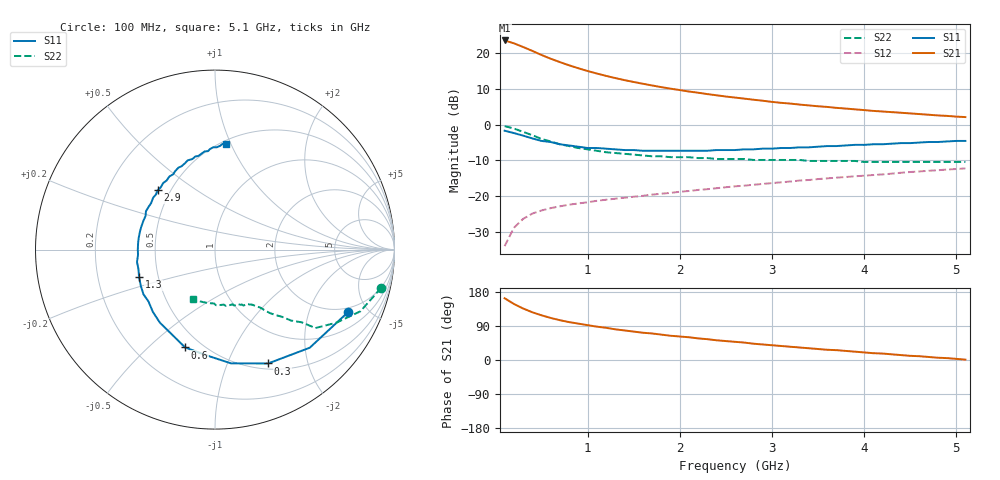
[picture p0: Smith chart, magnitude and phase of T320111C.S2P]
!AT-32011
!S PARAMETERS at Vce=1 V  Ic=5mA.  LAST UPDATED 01-05-95
# ghz s ma r 50
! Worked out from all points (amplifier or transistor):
!   51 points, 100 MHz to 5.1 GHz, reference 50 ohm
!   highest |S21| = 23.5 dB at 100 MHz (marker M1)
!   |S21| within 3 dB of that: start of sweep to 408.5 MHz
!   unconditionally stable (mu >= 1): 1.731 GHz to end of sweep
!   at 900 MHz: K = 0.67, MSG = 18.9 dB, |S12| = -22.0 dB
!   at 2.6 GHz: K = 1.12, MAG = 10.3 dB, |S12| = -17.3 dB
!   at 5.1 GHz: K = 1.02, MAG = 6.2 dB, |S12| = -12.3 dB
!   S11 on the Smith chart (normalised r, x): 100 MHz: 1.76, -3.73; 300 MHz: 0.57, -1.41; 600 MHz: 0.41, -0.66; 1.3 GHz: 0.39, -0.15; 2.9 GHz: 0.43, +0.36; 5.1 GHz: 0.53, +0.96
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0.1  0.82 -25.0  14.93 163.0  0.02 77.0  0.95 -13.0
0.2  0.76 -46.0  13.63 148.0  0.036 67.0  0.88 -23.0
0.3  0.7 -65.0  12.11 136.0  0.048 59.0  0.79 -31.0
0.4  0.64 -82.0  10.69 126.0  0.057 53.0  0.71 -38.0
0.5  0.59 -95.0  9.36 118.0  0.063 49.0  0.63 -40.0
0.6  0.57 -107.0  8.3 111.0  0.068 47.0  0.58 -43.0
0.7  0.53 -117.0  7.44 105.0  0.072 45.0  0.53 -45.0
0.8  0.51 -127.0  6.71 100.0  0.076 44.0  0.5 -47.0
0.9  0.49 -135.0  6.11 96.0  0.079 43.0  0.47 -49.0
1  0.47 -142.0  5.59 92.0  0.082 42.0  0.45 -50.0
1.1  0.47 -148.0  5.16 88.0  0.086 42.0  0.43 -51.0
1.3  0.45 -160.0  4.46 81.0  0.092 42.0  0.4 -53.0
1.4  0.44 -166.0  4.17 78.0  0.095 42.0  0.39 -54.0
1.6  0.43 -176.0  3.71 72.0  0.101 42.0  0.37 -56.0
1.8  0.43 175.0  3.33 67.0  0.108 42.0  0.36 -58.0
1.9  0.43 171.0  3.17 64.0  0.111 42.0  0.35 -60.0
2.2  0.43 158.0  2.78 57.0  0.122 42.0  0.34 -64.0
2.6  0.44 144.0  2.38 48.0  0.137 42.0  0.33 -69.0
2.9  0.46 134.0  2.15 41.0  0.148 41.0  0.32 -73.0
3.5  0.49 117.0  1.8 29.0  0.173 39.0  0.31 -82.0
4.3  0.54 98.0  1.49 15.0  0.206 35.0  0.3 -96.0
5.1  0.59 84.0  1.27 1.0  0.244 29.0  0.3 -114.0
